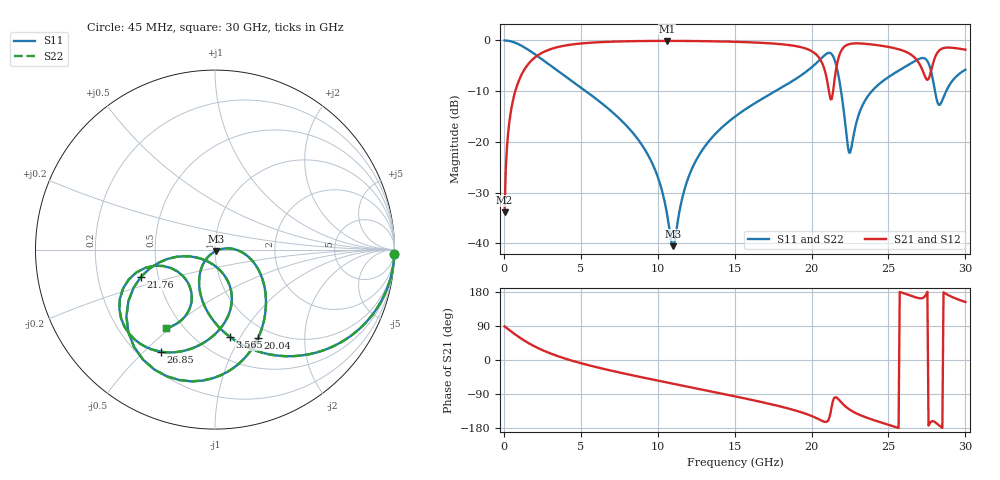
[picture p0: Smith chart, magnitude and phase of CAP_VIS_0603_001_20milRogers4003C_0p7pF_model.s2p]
! S-parameter model data by Modelithics Inc.  support@modelithics.com  813-866-6335  Tampa FL USA
! S-Parameter data specifications:
! Substrate: 20-mil Rogers 4003C, substrate thickness, H=0.508mm, Dielectric constant, Er=3.75
! PCB Mounting Pad Footprint: Pad width, PadW=0.90mm , Pad length, PadL=1.00mm , Pad gap, PadG (edge-to-edge)=1.00mm , Reference planes=3.0mm apart
! Created Wed Nov 18 13:16:51 2015
# hz S ma R 50
! 2 Port Network Data from SP1.SP block
! freq  magS11  angS11  magS21  angS21  magS12  angS12  magS22  angS22
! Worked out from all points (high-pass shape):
!   401 points, 45 MHz to 30 GHz, reference 50 ohm
!   highest |S21| = -0.09 dB at 10.6 GHz (marker M1); lowest = -33.9 dB at 45 MHz (marker M2)
!   |S21| within 3 dB of the highest: 2.13 GHz to 20.4 GHz (18.27 GHz wide, 162 % of centre); 21.79 GHz to 26.59 GHz (4.804 GHz wide, 19.9 % of centre)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
!   lowest |S11| = -40.5 dB at 10.98 GHz (marker M3), VSWR 1.02, Z = 50.4 - j0.866 ohm
!   |S11| at or under -10 dB: 5.33 GHz to 17.64 GHz (12.31 GHz wide, 107 % of centre); 21.92 GHz to 23.92 GHz (1.999 GHz wide, 8.72 % of centre); 28.03 GHz to 28.75 GHz (724.4 MHz wide, 2.55 % of centre)
!   |S22| runs from -40.5 to 0.0 dB; largest |S21 - S12| = 0
!   S11 on the Smith chart (normalised r, x): 45 MHz: 1, -81; 3.565 GHz: 0.70, -0.91; 20.04 GHz: 0.85, -1.20; 21.76 GHz: 0.40, -0.15; 26.85 GHz: 0.29, -0.56; 30 GHz: 0.41, -0.48
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4.5e7  0.9998 -1.4  0.02022 88.6  0.02022 88.6  0.9998 -1.4
4.194375e8  0.9826 -13.1  0.1854 76.9  0.1854 76.9  0.9826 -13.1
9.4365e8  0.9194 -28.5  0.3921 61.5  0.3921 61.5  0.9194 -28.5
3.564712e9  0.4943 -80.2  0.8648 9.3  0.8648 9.3  0.4943 -80.2
5.062462e9  0.3387 -98.1  0.935 -9.0  0.935 -9.0  0.3387 -98.1
8.357512e9  0.124 -126.9  0.9839 -40.4  0.9839 -40.4  0.124 -126.9
1.007992e10  0.04173 -132.9  0.9895 -55.0  0.9895 -55.0  0.04173 -132.9
1.060414e10  0.01946 -121.4  0.9898 -59.3  0.9898 -59.3  0.01946 -121.4
1.097858e10  0.009391 -66.2  0.9897 -62.4  0.9897 -62.4  0.009391 -66.2
1.240144e10  0.062 6.3  0.9866 -74.1  0.9866 -74.1  0.062 6.3
1.50225e10  0.1775 -10.0  0.9699 -95.9  0.9699 -95.9  0.1775 -10.0
2.003996e10  0.549 -64.2  0.7792 -148.3  0.7792 -148.3  0.549 -64.2
2.108839e10  0.7535 -105.2  0.3455 -158.9  0.3455 -158.9  0.7535 -105.2
2.176238e10  0.439 -159.8  0.682 -104.2  0.682 -104.2  0.439 -159.8
2.251125e10  0.07865 -107.9  0.9253 -131.8  0.9253 -131.8  0.07865 -107.9
2.34099e10  0.2454 -68.6  0.929 -149.5  0.929 -149.5  0.2454 -68.6
2.505742e10  0.4416 -86.3  0.8599 -171.7  0.8599 -171.7  0.4416 -86.3
2.685472e10  0.6436 -117.9  0.6378 164.3  0.6378 164.3  0.6436 -117.9
2.752871e10  0.6268 -148.2  0.4084 179.9  0.4084 179.9  0.6268 -148.2
2.797804e10  0.3469 -165.0  0.6504 -162.7  0.6504 -162.7  0.3469 -165.0
2.835248e10  0.2331 -133.5  0.8097 -174.6  0.8097 -174.6  0.2331 -133.5
3e10  0.5152 -121.7  0.8112 153.1  0.8112 153.1  0.5152 -121.7
